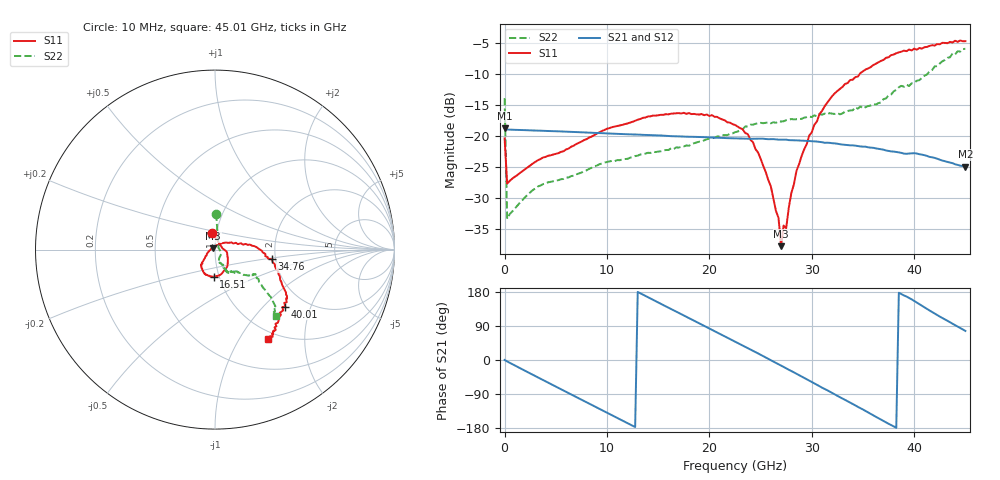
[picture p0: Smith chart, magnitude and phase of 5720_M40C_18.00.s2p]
! Device:  ADRF5720
! Description: 0.5dB LSB GaAs MMIC 6-bit Digital Attenuator
! Frequency:  0.000009 -  40 GHz
! Ports:
!	RF1	= Port 1
!	RF2	= Port 2
! Vdd:  3.3 Volt
! Vss:  -3.3 Volt
! Control:  0/3.3 Volt
! State:  18.00 dB attenuation
! Data:  The device was measured using G-S-G Probes on a matrix board.
!  Data was collected using an calibrated 4 port network analyzer.
!  The reference plane for this measurement is at the launchers.
! Note:  Analog Devices supplies this data as a sample of measured data
!  for this product.  Your particular data for this product may vary.
!  Data was taken at -40 degrees C.
!  Analog Devices reserves the right to change this data at anytime.
# GHZ S DB R 45.0
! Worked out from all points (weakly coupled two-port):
!   181 points, 10 MHz to 45.01 GHz, reference 45 ohm
!   highest |S21| = -18.83 dB at 10 MHz (marker M1); lowest = -25.0 dB at 45.01 GHz (marker M2)
!   lowest |S11| = -37.8 dB at 27.01 GHz (marker M3), VSWR 1.03, Z = 44.1 + j0.671 ohm
!   |S11| at or under -10 dB: start of sweep to 34.72 GHz
!   |S22| runs from -33.4 to -6.0 dB; largest |S21 - S12| = 0.00041
!   S11 on the Smith chart (normalised r, x): 10 MHz: 0.96, +0.18; 16.51 GHz: 0.94, -0.29; 34.76 GHz: 1.90, -0.23; 40.01 GHz: 1.58, -1.35; 45.01 GHz: 0.90, -1.34
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0.01  -20.43 98.5  -18.83 0.1  -18.86 0.1  -13.96 88.2
0.26  -27.74 12.9  -19.01 -3.8  -19.04 -3.9  -33.41 22.2
3.26  -23.96 -8.8  -19.19 -45.9  -19.21 -46.0  -28.20 -28.5
7.76  -20.72 -38.6  -19.47 -108.1  -19.49 -108.2  -25.75 -61.7
15.26  -16.64 -84.3  -19.97 148.4  -19.99 148.3  -22.52 -71.5
16.51  -16.42 -92.5  -20.09 131.2  -20.11 131.2  -22.17 -69.5
20.26  -16.69 -114.0  -20.30 79.5  -20.32 79.4  -20.40 -63.6
22.76  -18.52 -131.4  -20.44 45.1  -20.46 45.0  -19.35 -64.2
24.26  -21.03 -136.8  -20.50 24.4  -20.53 24.4  -18.23 -62.7
25.51  -25.86 -152.6  -20.54 6.4  -20.57 6.3  -17.93 -61.7
26.76  -33.27 160.5  -20.64 -11.2  -20.66 -11.4  -17.69 -61.3
27.01  -37.83 143.6  -20.64 -14.7  -20.66 -14.8  -17.72 -62.9
27.26  -34.51 119.5  -20.64 -18.3  -20.66 -18.4  -17.68 -61.3
27.51  -34.92 75.1  -20.64 -22.0  -20.66 -22.1  -17.50 -62.4
28.01  -29.28 50.5  -20.73 -29.0  -20.75 -29.1  -17.32 -62.9
28.51  -25.69 42.6  -20.76 -36.2  -20.79 -36.3  -17.35 -62.4
30.26  -18.23 18.1  -20.92 -61.7  -20.95 -61.8  -16.71 -61.0
32.01  -13.59 5.8  -21.22 -87.1  -21.24 -87.3  -16.45 -56.0
34.76  -9.90 -9.6  -21.74 -127.1  -21.77 -127.3  -15.27 -48.7
37.76  -7.01 -29.9  -22.54 -171.7  -22.56 -171.9  -13.36 -40.8
40.01  -5.95 -39.0  -22.83 155.8  -22.85 155.7  -11.49 -32.8
45.01  -4.76 -59.0  -24.98 76.7  -25.00 76.6  -5.98 -47.2
